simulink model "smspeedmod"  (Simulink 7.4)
settings: Solver=ode23t  StartTime=0.0  StopTime=50  MaxStep=0.05  RelTol=1e-3  AbsTol=1e-3
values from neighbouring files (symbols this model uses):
  Bm = 0.10    (= 0.1)    [IMabc2.m]    (also in imabcparam.m = 0.01; IMabcrun0.m = 0.01; IMabcrun1.m = 0.001; IMcur0.m = 1e-06)
  H = 0.60    (= 0.6)    [IMabc2.m]    (also in IMcur0.m = 0.3; imdef0vec.m = 0.3; imdef1vec.m = 0.3; imdef2vec.m = 0.3)
  Ra = .95    (= 0.95)    [altwdgs.m]    (also in Ccurverun.m = 0.018)
  wo = 2*pi*freq0    [calc0.m]    (also in IMabc2.m = 376.991118431; imabcparam.m = 376.991118431; IMabcrun0.m = 376.991118431; IMabcrun1.m = 376.991118431)
undefined symbols (not defined in the file or in its folder): fa0, fk0, Lal, Lfl, Lkdl, Lkql, Lmd, Lmq, phif0, Rf, Rkd, Rkq, vf0

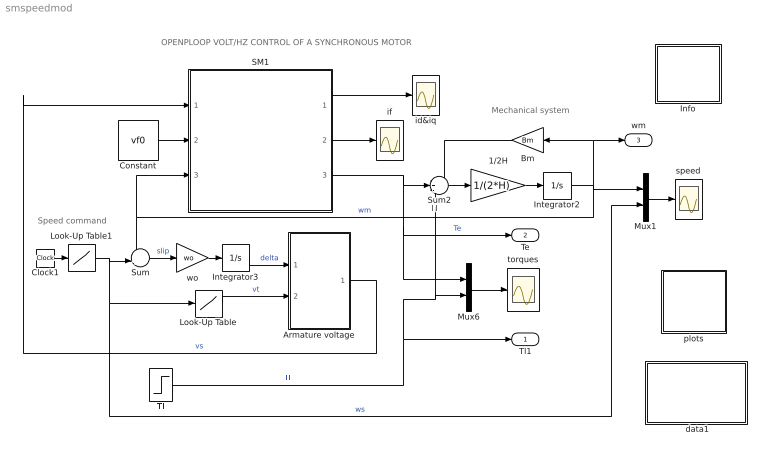
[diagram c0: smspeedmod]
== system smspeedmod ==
  note: Tl
  note: OPENPLOOP VOLT/HZ CONTROL OF A SYNCHRONOUS MOTOR
  note: Mechanical system
  note: Speed command
  " data1" : Subsystem
  1/2H : Gain  Gain=1/(2*H)  ParameterDataType=sfix(16)  ParameterScaling=2^0  OutDataType=sfix(16)  OutScaling=2^0
  Armature voltage : Subsystem
  Bm : Gain  Gain=Bm  ParameterDataType=sfix(16)  ParameterScaling=2^0  OutDataType=sfix(16)  OutScaling=2^0
  Clock1 : Clock
  Constant : Constant  Value=vf0  OutDataType=sfix(16)  OutScaling=2^0
  Info : Subsystem
  Integrator2 : Integrator
  Integrator3 : Integrator
  Look-Up Table : Lookup  InputValues=[-1 0 1]  Table=[1 0.04 1]  OutDataType=sfix(16)  OutScaling=2^0
  Look-Up Table1 : Lookup  InputValues="[0  15 35 45 50]"  Table="[0  1 1 0.8 0.8]"  OutDataType=sfix(16)  OutScaling=2^0
  Mux1 : Mux  Inputs=2
  Mux6 : Mux  Inputs=2
  SM1 : Subsystem
  Sum : Sum  Inputs=-+|  OutDataType=sfix(16)  OutScaling=2^0
  Sum2 : Sum  Inputs=-+-  OutDataType=sfix(16)  OutScaling=2^0
  Tl : Step  Time=25  After=0.6  SampleTime=0
  id&iq : Scope
  if : Scope
  plots : Subsystem
  speed : Scope
  torques : Scope
  wo : Gain  Gain=wo  ParameterDataType=sfix(16)  ParameterScaling=2^0  OutDataType=sfix(16)  OutScaling=2^0
  Tl1 : Outport
  Te : Outport  Port=2
  wm : Outport  Port=3
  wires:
  1/2H/1 -> Integrator2/1
  Bm/1 -> Sum2/1
  SM1/3(Te) -> Sum2/2, Mux6/1, Te/1  "Te"
  Sum/1 -> wo/1  "slip"
  wo/1 -> Integrator3/1
  Integrator3/1 -> Armature voltage/1(delta)  "delta"
  Integrator2/1 -> Sum/1, SM1/3(wm), Bm/1, wm/1, Mux1/1  "wm"
  Tl/1 -> Mux6/2, Sum2/3, Tl1/1  "Tl"
  Look-Up Table/1 -> Armature voltage/2(Vt)  "vt"
  Look-Up Table1/1 -> Sum/2, Look-Up Table/1, Mux1/2  "ws"
  Armature voltage/1(vs) -> SM1/1(vs)  "vs"
  SM1/2(if) -> if/1
  Mux6/1 -> torques/1
  SM1/1(ia) -> id&iq/1
  Sum2/1 -> 1/2H/1
  Clock1/1 -> Look-Up Table1/1
  Mux1/1 -> speed/1
  Constant/1 -> SM1/2(vf)

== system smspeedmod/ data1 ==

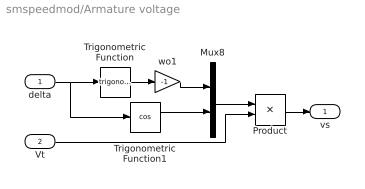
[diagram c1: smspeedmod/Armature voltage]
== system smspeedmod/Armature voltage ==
  delta : Inport  OutDataType=sfix(16)  OutScaling=2^0
  Vt : Inport  Port=2  OutDataType=sfix(16)  OutScaling=2^0
  Mux8 : Mux  Inputs=2
  Product : Product  OutDataType=sfix(16)  OutScaling=2^0
  Trigonometric Function : Trigonometry
  Trigonometric Function1 : Trigonometry  Operator=cos
  wo1 : Gain  Gain=-1  ParameterDataType=sfix(16)  ParameterScaling=2^0  OutDataType=sfix(16)  OutScaling=2^0
  vs : Outport
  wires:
  delta/1 -> Trigonometric Function/1, Trigonometric Function1/1
  Trigonometric Function/1 -> wo1/1
  Mux8/1 -> Product/1
  wo1/1 -> Mux8/1
  Trigonometric Function1/1 -> Mux8/2
  Product/1 -> vs/1
  Vt/1 -> Product/2

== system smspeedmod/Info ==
  note: Open-loop Volt/Hz control of a synchronous motor
  note: First double click DATA block , change parameters if required, and initialize to establish IC, then RUN.

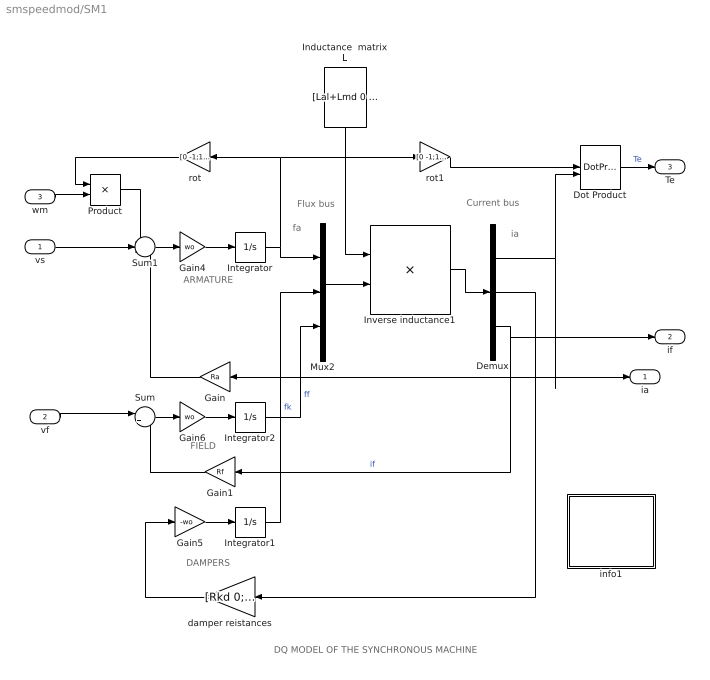
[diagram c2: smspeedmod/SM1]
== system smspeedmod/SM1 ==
  note: DAMPERS
  note: ARMATURE
  note: fa
  note: ia
  note: FIELD
  note: DQ MODEL OF THE SYNCHRONOUS MACHINE
  note: Flux bus
  note: Current bus
  vs : Inport  OutDataType=sfix(16)  OutScaling=2^0
  vf : Inport  Port=2  OutDataType=sfix(16)  OutScaling=2^0
  wm : Inport  Port=3  OutDataType=sfix(16)  OutScaling=2^0
  Demux : Demux  Outputs=3
  Dot Product : DotProduct  OutDataType=fixdt(1, 16)  OutScaling=2^-10
  Gain : Gain  Gain=Ra  ParameterDataType=sfix(16)  ParameterScaling=2^0  OutDataType=sfix(16)  OutScaling=2^0
  Gain1 : Gain  Gain=Rf  ParameterDataType=sfix(16)  ParameterScaling=2^0  OutDataType=sfix(16)  OutScaling=2^0
  Gain4 : Gain  Gain=wo  ParameterDataType=sfix(16)  ParameterScaling=2^0  OutDataType=sfix(16)  OutScaling=2^0
  Gain5 : Gain  Gain=-wo  ParameterDataType=sfix(16)  ParameterScaling=2^0  OutDataType=sfix(16)  OutScaling=2^0
  Gain6 : Gain  Gain=wo  ParameterDataType=sfix(16)  ParameterScaling=2^0  OutDataType=sfix(16)  OutScaling=2^0
  Inductance  matrix L : Constant  Value=[Lal+Lmd 0 Lmd 0 Lmd;0 Lal+Lmq 0 Lmq 0;Lmd 0 Lmd+Lkdl 0 Lmd;0 Lmq 0 Lmq+Lkql 0;Lmd 0 Lmd 0 Lmd+Lfl]  VectorParams1D=off  OutDataType=fixdt(1, 16)  OutScaling=2^0
  Integrator : Integrator  InitialCondition=fa0
  Integrator1 : Integrator  InitialCondition=fk0
  Integrator2 : Integrator  InitialCondition=phif0
  Inverse inductance1 : Product  Inputs=/*  Multiplication=Matrix(*)  OutDataType=sfix(16)  OutScaling=2^0
  Mux2 : Mux  Inputs=3
  Product : Product  OutDataType=sfix(16)  OutScaling=2^0
  Sum : Sum  Inputs=|+-  OutDataType=sfix(16)  OutScaling=2^0
  Sum1 : Sum  Inputs=-+-  OutDataType=sfix(16)  OutScaling=2^0
  damper reistances : Gain  Gain=[Rkd 0;0 Rkq]  Multiplication=Matrix(K*u)  ParameterDataType=sfix(16)  ParameterScaling=2^0  OutDataType=sfix(16)  OutScaling=2^0
  info1 : Subsystem
  rot : Gain  Gain=[0 -1;1 0]  Multiplication=Matrix(K*u)  ParameterDataType=sfix(16)  ParameterScaling=2^0  OutDataType=sfix(16)  OutScaling=2^0
  rot1 : Gain  Gain=[0 -1;1 0]  Multiplication=Matrix(K*u)  ParameterDataType=sfix(16)  ParameterScaling=2^0  OutDataType=sfix(16)  OutScaling=2^0
  ia : Outport
  if : Outport  Port=2
  Te : Outport  Port=3
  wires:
  Product/1 -> Sum1/1
  rot/1 -> Product/1
  wm/1 -> Product/2
  Gain5/1 -> Integrator1/1
  damper reistances/1 -> Gain5/1
  Integrator/1 -> Mux2/1, rot/1, rot1/1
  Sum1/1 -> Gain4/1
  Gain4/1 -> Integrator/1
  vs/1 -> Sum1/2
  Gain/1 -> Sum1/3
  Gain6/1 -> Integrator2/1
  Sum/1 -> Gain6/1
  vf/1 -> Sum/1
  Gain1/1 -> Sum/2
  rot1/1 -> Dot Product/1
  Demux/1 -> Gain/1, ia/1, Dot Product/2
  Integrator1/1 -> Mux2/2  "fk"
  Integrator2/1 -> Mux2/3  "ff"
  Demux/2 -> damper reistances/1
  Demux/3 -> if/1, Gain1/1  "if"
  Dot Product/1 -> Te/1  "Te"
  Mux2/1 -> Inverse inductance1/2
  Inverse inductance1/1 -> Demux/1
  Inductance  matrix L/1 -> Inverse inductance1/1

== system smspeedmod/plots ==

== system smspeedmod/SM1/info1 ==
  note: Synchronous machine transients under shortcircuit
  note: This demonstration illustrates the dynamics of a synchronous generator, initially at no load, following a three-phase short circuit at the terminals.
